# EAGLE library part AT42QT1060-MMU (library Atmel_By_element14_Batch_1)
QTOUCH 6-CHANNEL SENSOR IC
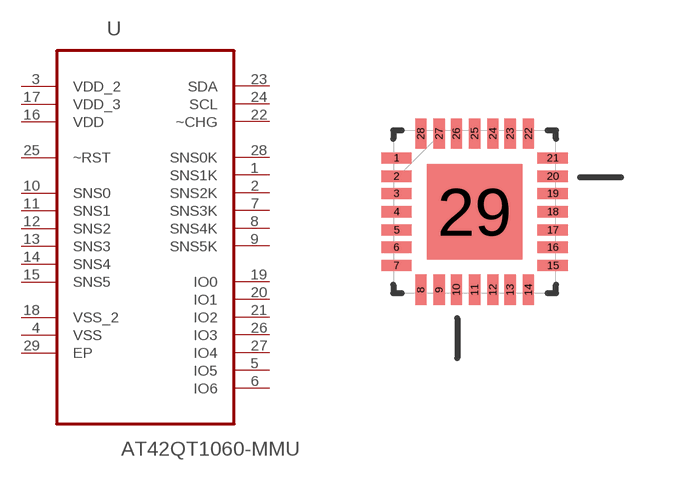
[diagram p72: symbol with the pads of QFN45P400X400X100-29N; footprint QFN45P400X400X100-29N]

Designator prefix U

## AT42QT1060-MMU (MPN: AT42QT1060-MMU; OC_FARNELL: 1748489; OC_NEWARK: 68T4659; PACKAGE: QFN-28; SUPPLIER: ATMEL)  [QFN45P400X400X100-29N]
1  SNS1K
2  SNS2K
3  VDD_2  pwr
4  VSS  pas
5  IO5
6  IO6
7  SNS3K
8  SNS4K
9  SNS5K
10  SNS0
11  SNS1
12  SNS2
13  SNS3
14  SNS4
15  SNS5
16  VDD  pwr
17  VDD_3  pwr
18  VSS_2  pas
19  IO0
20  IO1
21  IO2
22  ~CHG  out
23  SDA  out
24  SCL  out
25  ~RST  in
26  IO3
27  IO4
28  SNS0K
29  EP  pas

## Footprint QFN45P400X400X100-29N (pad centres in mm)
smd 0.762 x 0.279: 1 -1.956,1.346; 2 -1.956,0.889; 3 -1.956,0.457; 4 -1.956,0; 5 -1.956,-0.457; 6 -1.956,-0.889; 7 -1.956,-1.346; 15 1.956,-1.346; 16 1.956,-0.889; 17 1.956,-0.457; 18 1.956,0; 19 1.956,0.457; 20 1.956,0.889; 21 1.956,1.346
smd 0.279 x 0.762: 8 -1.346,-1.956; 9 -0.889,-1.956; 10 -0.457,-1.956; 11 0,-1.956; 12 0.457,-1.956; 13 0.889,-1.956; 14 1.346,-1.956; 22 1.346,1.956; 23 0.889,1.956; 24 0.457,1.956; 25 0,1.956; 26 -0.457,1.956; 27 -0.889,1.956; 28 -1.346,1.956
smd 2.388 x 2.388: 29 0,0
